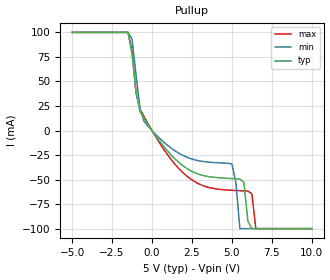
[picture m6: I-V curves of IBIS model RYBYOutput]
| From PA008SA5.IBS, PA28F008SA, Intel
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|****************Ready/Busy Output Model*****************************
[Model]   RYBYOutput
Model_type   Output
|   For RY/BY# pin 36
Vinl = 0.8V
Vinh = 2.0V
| Variable   typ   min   max
C_comp   9.61p   NA   11.6p
[Voltage Range]   5.0V   4.5V   5.5V
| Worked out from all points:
|   slope of the pullup table from 0 to 0.75 V, typ, clamps not added: 45.2 ohm
[Pulldown]
| [Pullup] and [Pulldown] IV curves include only the current through
| the channels of output driver transistors when outputs are enabled
| with OE# = VIL.  Although the output driver transistors have np and
| pn diodes inherently created by CMOS IC fabrication between the
| drain and bulk of n-channel and p-channel CMOS transistors,
| the current through these junction diodes is not included in
| [Pullup] or [Pulldown].  Instead that drain/bulk diode current is
| included in the [POWER_clamp] or [GND_clamp] sections, which are
| not dependent on the state of OE# or output data value.  The RY/BY#
| Pulldown information is not provided for this device.  The table
| below is for the compatibility with some IBIS parsers.
|Voltage   I(typ)   I(min)   I(max)
-5V       0A         0A         0A
0V        0A         0A         0A
5V        0A         0A         0A
10V       0A         0A         0A
[GND_clamp]
| The RY/BY# pin is always active and does NOT float to tri-state when
| the chip is deselected or when the data outputs are disabled.
| Therefore, the table below is included for the compatibility with
| some IBIS parsers.
|Voltage   I(typ)   I(min)   I(max)
-5V       0A         0A         0A
0V        0A         0A         0A
5V        0A         0A         0A
10V       0A         0A         0A
[Pullup]
| (Voltages for [Pullup] and [POWER_clamp] are specified with
| negative respect to Vcc.  Reference the IBIS documentation
| for more information regarding Vtable = Vcc - Voutput.
| This method keeps -Vds constant for the values in all three
| columns across a line of the table.)
| [Pullup] and [Pulldown] IV curves include only the current through
| the channels of output driver transistors when outputs are enabled
| with OE# = VIL.  Although the output driver transistors have np and
| pn diodes inherently created by CMOS IC fabrication between the
| drain and bulk of n-channel and p-channel CMOS transistors,
| the current through these junction diodes is not included in
| [Pullup] or [Pulldown].  Instead that drain/bulk diode current is
| included in the [POWER_clamp] or [GND_clamp] sections, which are
| not dependent on the state of OE# or output data value.
|Voltage  I(typ)   I(min)   I(max)
-5V       100mA      100mA      100mA
-1.5V     100mA      100mA      100mA
-1.25V    78.12mA    93.3mA     81.44mA
-750mV    19.27mA    22.34mA    21.94mA
500mV     -11.29mA   -8.256mA   -13.25mA
2.5V      -41.55mA   -28.99mA   -50.24mA
5V        -48.82mA   -34.02mA   -60.8mA
5.25V     -49.02mA   -52.99mA   -61.02mA
5.5V      -49.27mA   -99.85mA   -61.2mA
6.25V     -99.85mA   -99.85mA   -64.38mA
6.5V      -99.85mA   -99.85mA   -99.85mA
10V       -99.85mA   -99.85mA   -99.85mA
[POWER_clamp]
| The RY/BY# pin is always active and does NOT float to tri-state when
| the chip is deselected or when the data outputs are disabled.
| Therefore, the table below is included for the compatibility with
| some IBIS parsers.
|Voltage  I(typ)   I(min)   I(max)
-5V       0A         0A         0A
0V        0A         0A         0A
5V        0A         0A         0A
10V       0A         0A         0A
[Ramp]
| The RY/BY# Ramp information is not provided for this device.  The table
| below is for the compatibility with some IBIS parsers.
| Variable   typ   min   max
 dV/dt_r   0V/0ns   0V/0ns   0V/0ns
 dV/dt_f   0V/0ns   0V/0ns   0V/0ns
